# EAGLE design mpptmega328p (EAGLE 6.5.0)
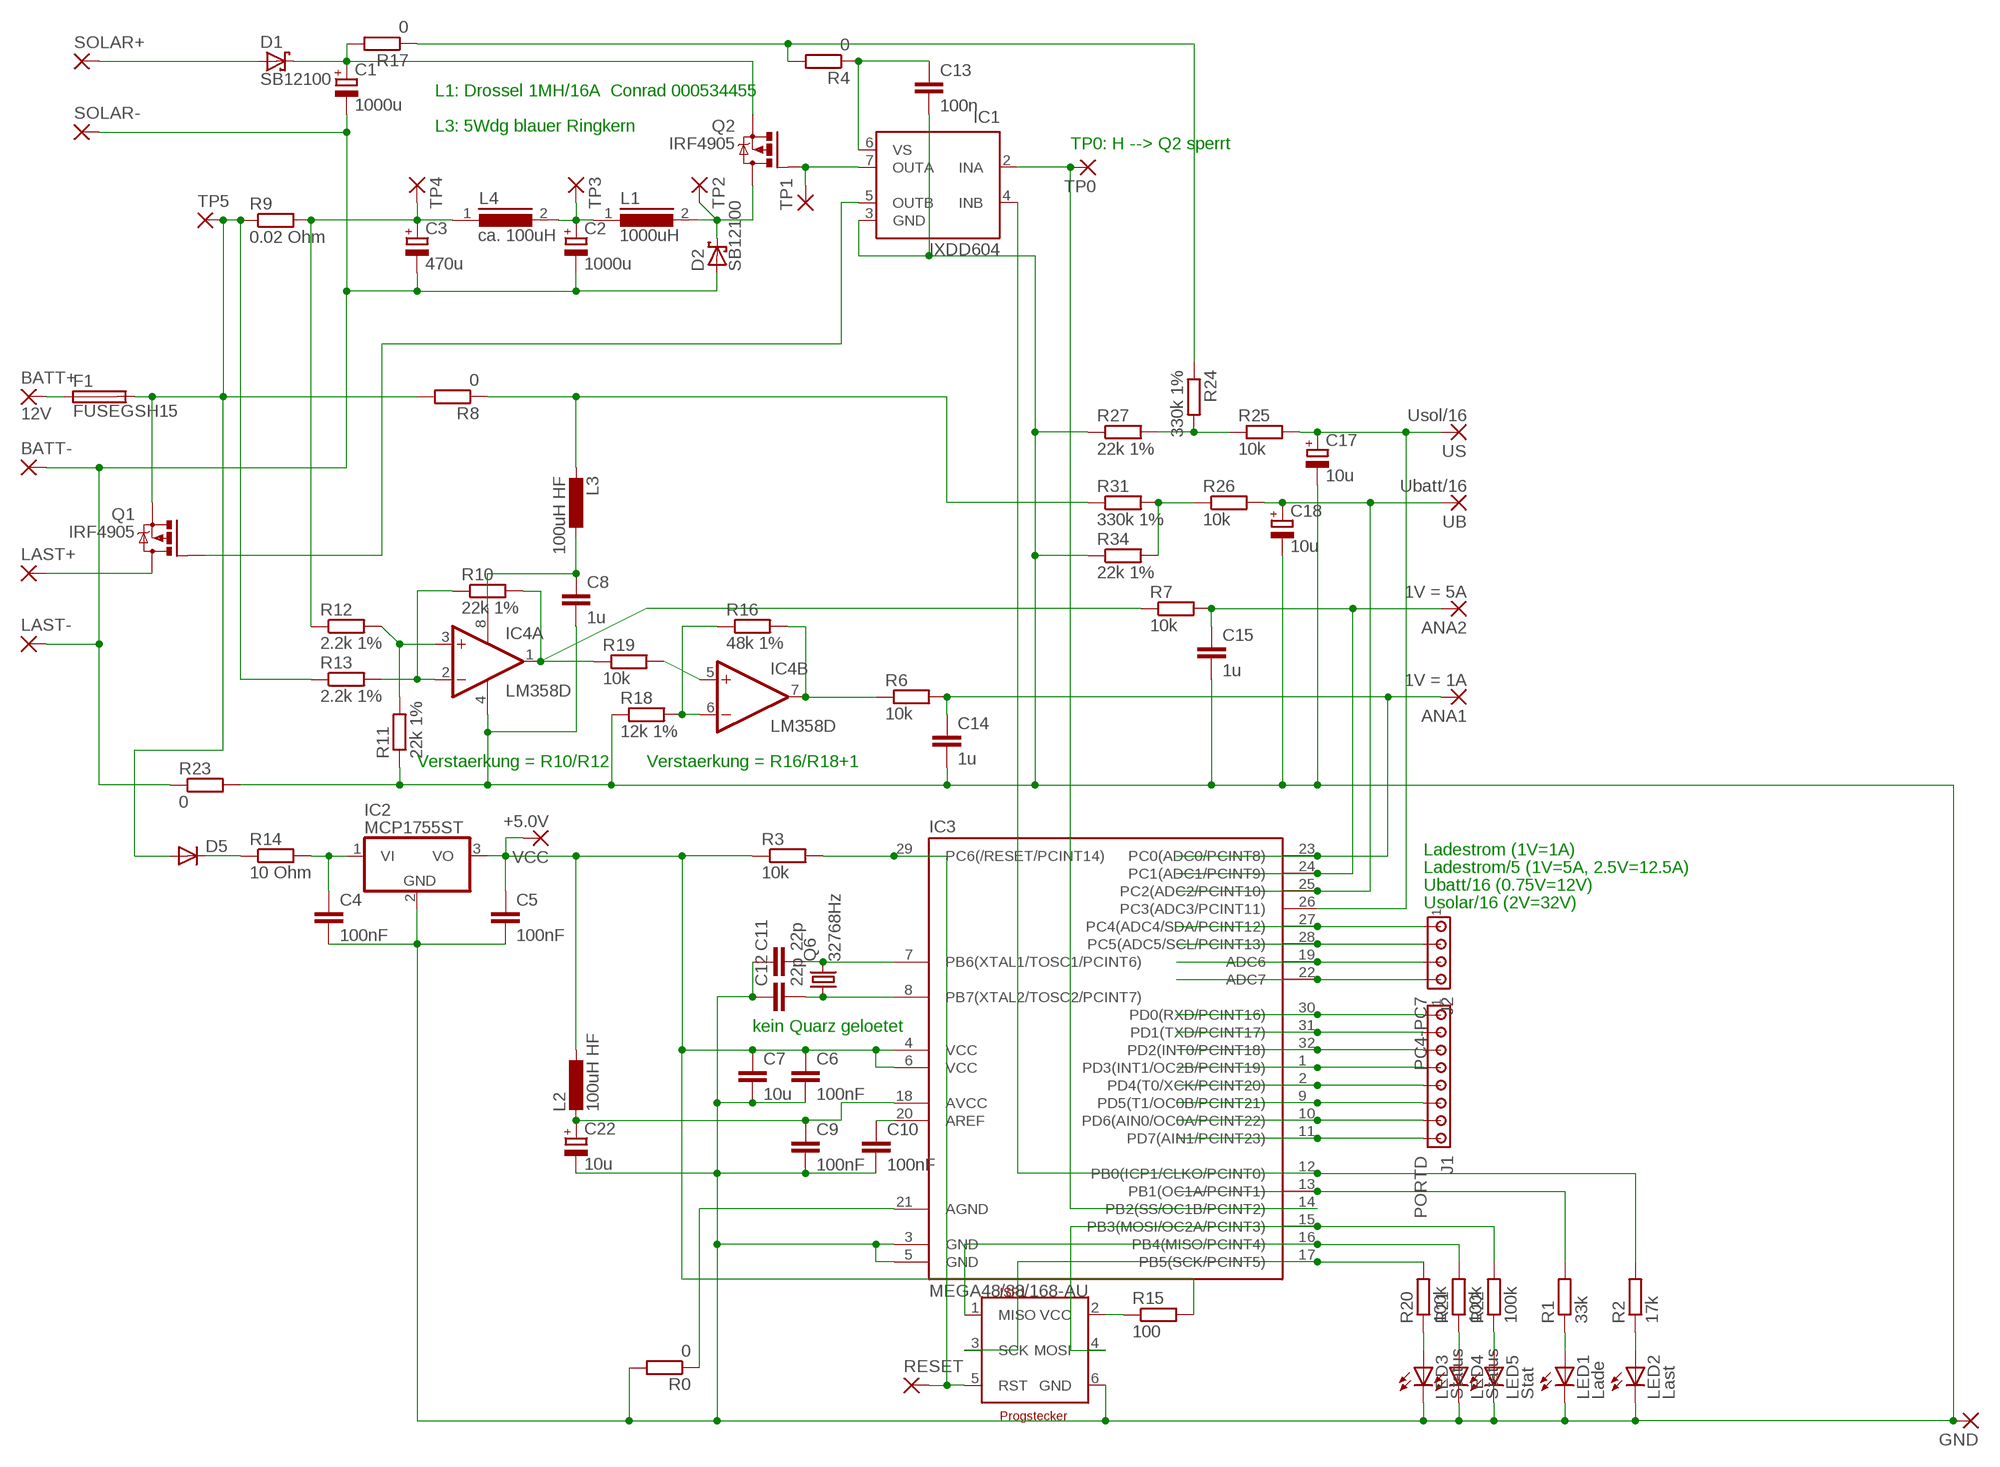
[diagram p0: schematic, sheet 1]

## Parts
ANA1  1V = 1A  WIREPAD1,6/0,8  [1,6/0,8]
ANA2  1V = 5A  WIREPAD1,6/0,8  [1,6/0,8]
BATT+  12V  WIREPAD3,81/1,1  [3,81/1,1]
BATT-  WIREPAD3,81/1,1  [3,81/1,1]
C1  1000u  CPOL-EUE5-13  [E5-13]
C2  1000u  CPOL-EUE5-13  [E5-13]
C3  470u  CPOL-EUE3.5-10  [E3,5-10]
C4  100nF  C-EUC1206  [C1206]
C5  100nF  C-EUC1206  [C1206]
C6  100nF  C-EUC1206K  [C1206K]
C7  10u  C-EUC1206  [C1206]
C8  1u  C-EUC1206K  [C1206K]
C9  100nF  C-EUC1206K  [C1206K]
C10  100nF  C-EUC1206K  [C1206K]
C11  22p  C-EU025-024X044  [C025-024X044]
C12  22p  C-EU025-024X044  [C025-024X044]
C13  100n  C-EUC1206K  [C1206K]
C14  1u  C-EU025-025X050  [C025-025X050]
C15  1u  C-EU025-025X050  [C025-025X050]
C17  10u  CPOL-EUE2-5  [E2-5]
C18  10u  CPOL-EUE2-5  [E2-5]
C22  10u  CPOL-EUE2.5-5  [E2,5-5]
D1  SB12100  1N5908  [C4111-15]
D2  SB12100  1N5908  [C4111-15]
D5  1N4004  [DO41-10]
F1  FUSEGSH15  [GSH15]
GND  WIREPAD2,15/1,0  [2,15/1,0]
IC1  IXDD604  IR4427S  [SO08]
IC2  MCP1755ST  MCP1703DB  [SOT223]
IC3  MEGA48/88/168-AU  [TQFP32-08]
IC4  LM358D  [SO08]
ISP1  Progstecker  ISP6N  [ISP6]
J1  PORTD  MTA08-100  [10X08MTA]
J2  PC4-PC7  MTA04-100  [10X04MTA]
L1  1000uH  A26GFC  [A26GFC]
L2  100uH HF  L-EU0204/7  [0204/7]
L3  100uH HF  L-EU0204/7  [0204/7]
L4  ca. 100uH  82114R  [82114R]
LAST+  WIREPAD3,81/1,1  [3,81/1,1]
LAST-  WIREPAD3,81/1,1  [3,81/1,1]
LED1  Lade  LEDSFH482  [SFH482]
LED2  Last  LEDSFH482  [SFH482]
LED3  Status  LEDSFH482  [SFH482]
LED4  Status  LEDSFH482  [SFH482]
LED5  Stat  LEDSFH482  [SFH482]
Q1  IRF4905  IRF9530  [TO220BV]
Q2  IRF4905  IRF9530  [TO220BV]
Q6  32768Hz  CRYSTALTC26V  [TC26V]
R0  0  R-EU_R1206  [R1206]
R1  33k  R-EU_0204/2V  [0204V@1]
R2  17k  R-EU_0204/2V  [0204V@1]
R3  10k  R-EU_M1406  [M1406]
R4  0  R-EU_R1206  [R1206]
R6  10k  R-EU_0204/2V  [0204V@1]
R7  10k  R-EU_0204/2V  [0204V@1]
R8  0  R-EU_R1206  [R1206]
R9  0.02 Ohm  R-EU_0204/7  [0204/7@1]
R10  22k 1%  R-EU_0204/2V  [0204V@1]
R11  22k 1%  R-EU_0204/2V  [0204V@1]
R12  2.2k 1%  R-EU_0204/7  [0204/7@1]
R13  2.2k 1%  R-EU_0204/7  [0204/7@1]
R14  10 Ohm  R-EU_0204/5  [0204/5@1]
R15  100  R-EU_0204/5  [0204/5@1]
R16  48k 1%  R-EU_0204/2V  [0204V@1]
R17  0  R-EU_R1206  [R1206]
R18  12k 1%  R-EU_0204/5  [0204/5@1]
R19  10k  R-EU_0204/5  [0204/5@1]
R20  100k  R-EU_0204/2V  [0204V@1]
R21  100k  R-EU_0204/2V  [0204V@1]
R22  100k  R-EU_0204/2V  [0204V@1]
R23  0  R-EU_R1206  [R1206]
R24  330k 1%  R-EU_0204/7  [0204/7@1]
R25  10k  R-EU_0204/5  [0204/5@1]
R26  10k  R-EU_0204/5  [0204/5@1]
R27  22k 1%  R-EU_0204/5  [0204/5@1]
R31  330k 1%  R-EU_0204/7  [0204/7@1]
R34  22k 1%  R-EU_0204/5  [0204/5@1]
RESET  WIREPAD1,6/0,8  [1,6/0,8]
SOLAR+  WIREPAD3,81/1,1  [3,81/1,1]
SOLAR-  WIREPAD3,81/1,1  [3,81/1,1]
TP0  WIREPAD1,6/0,8  [1,6/0,8]
TP1  WIREPAD2,15/1,0  [2,15/1,0]
TP2  WIREPAD2,15/1,0  [2,15/1,0]
TP3  WIREPAD2,15/1,0  [2,15/1,0]
TP4  WIREPAD2,15/1,0  [2,15/1,0]
TP5  WIREPAD2,15/1,0  [2,15/1,0]
UB  Ubatt/16  WIREPAD2,15/1,0  [2,15/1,0]
US  Usol/16  WIREPAD2,15/1,0  [2,15/1,0]
VCC  +5.0V  WIREPAD2,54/0,9  [2,54/0,9]

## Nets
AGND [duenn]: IC3.21(AGND) R0.1
AVCC [duenn]: C9.1 C22.+ IC3.18(AVCC) L2.2
GND [dick]: C4.2 C5.2 C6.2 C7.2 C8.2 C9.2 C10.2 C11.1 C12.1 C13.2 C14.2 C15.2 C17.- C18.- C22.- GND.1(P) IC1.3(GND) IC2.2(GND) IC3.3(GND) IC3.5(GND) IC4.4(P:V-) ISP1.6(GND) LED1.K(C) LED2.K(C) LED3.K(C) LED4.K(C) LED5.K(C) R0.2 R11.1 R18.1 R23.2 R27.1 R34.1
GND2 [sehrdick]: BATT-.1(P) C1.- C2.- C3.- D2.A LAST-.1(P) R23.1 SOLAR-.1(P)
N$1 [dick]: LED1.A R1.1
N$2: IC1.4(INB) IC3.12(PB0(ICP1/CLKO/PCINT0)) R2.2
N$3: IC3.17(PB5(SCK/PCINT5)) ISP1.3(SCK) R20.2
N$4: IC3.13(PB1(OC1A/PCINT1)) R1.2
N$5 [dick]: LED2.A R2.1
N$6 [duenn]: C17.+ IC3.26(PC3(ADC3/PCINT11)) R25.2 US.1(P)
N$7: IC1.2(INA) IC3.14(PB2(SS/OC1B/PCINT2)) TP0.1(P)
N$8 [duenn]: IC1.5(OUTB) Q1.G
N$9 [duenn]: C18.+ IC3.25(PC2(ADC2/PCINT10)) R26.2 UB.1(P)
N$10: C10.1 IC3.20(AREF)
N$11: ISP1.2(VCC) R15.1
N$12 [duenn]: ANA2.1(P) C15.1 IC3.24(PC1(ADC1/PCINT9)) R7.2
N$13 [duenn]: ANA1.1(P) C14.1 IC3.23(PC0(ADC0/PCINT8)) R6.2
N$14 [dick]: D5.C R14.1
N$15: IC3.27(PC4(ADC4/SDA/PCINT12)) J2.1
N$16: IC3.28(PC5(ADC5/SCL/PCINT13)) J2.2
N$17: IC3.19(ADC6) J2.3
N$18 [dick]: C4.1 IC2.1(VI) R14.2
N$19: IC3.22(ADC7) J2.4
N$20 [sehrdick]: BATT+.1(P) F1.1
N$21 [sehrdick]: D1.A SOLAR+.1(P)
N$24 [sehrdick]: D2.C L1.2 Q2.D TP2.1(P)
N$25: IC3.16(PB4(MISO/PCINT4)) ISP1.1(MISO) R21.2
N$26: IC3.29(PC6(/RESET/PCINT14)) ISP1.5(RST) R3.2 RESET.1(P)
N$27: IC3.15(PB3(MOSI/OC2A/PCINT3)) ISP1.4(MOSI) R22.2
N$28 [dick]: IC1.7(OUTA) Q2.G TP1.1(P)
N$29 [sehrdick]: C2.+ L1.1 L4.2 TP3.1(P)
N$31 [dick]: LED3.A R20.1
N$32 [duenn]: IC4.2(A:-IN) R10.1 R13.2
N$33 [dick]: LED4.A R21.1
N$34 [dick]: LED5.A R22.1
N$35: C11.2 IC3.7(PB6(XTAL1/TOSC1/PCINT6)) Q6.2
N$36: C12.2 IC3.8(PB7(XTAL2/TOSC2/PCINT7)) Q6.1
N$37 [duenn]: IC4.3(A:+IN) R11.2 R12.2
N$38 [dick]: L3.2 R8.1 R31.1
N$39 [duenn]: IC4.6(B:-IN) R16.1 R18.2
N$40 [duenn]: IC4.5(B:+IN) R19.2
N$42 [duenn]: IC4.7(B:OUT) R6.1 R16.2
N$43 [sehrdick]: LAST+.1(P) Q1.D
N$47 [duenn]: IC4.1(A:OUT) R7.1 R10.2 R19.1
N$50: IC3.30(PD0(RXD/PCINT16)) J1.1
N$51: IC3.31(PD1(TXD/PCINT17)) J1.2
N$52: IC3.32(PD2(INT0/PCINT18)) J1.3
N$53: IC3.1(PD3(INT1/OC2B/PCINT19)) J1.4
N$54: IC3.2(PD4(T0/XCK/PCINT20)) J1.5
N$55: IC3.9(PD5(T1/OC0B/PCINT21)) J1.6
N$56: IC3.10(PD6(AIN0/OC0A/PCINT22)) J1.7
N$57: IC3.11(PD7(AIN1/PCINT23)) J1.8
N$58 [duenn]: R24.2 R25.1 R27.2
N$60 [sehrdick]: C3.+ L4.1 R9.2 R12.1 TP4.1(P)
N$64 [duenn]: R26.1 R31.2 R34.2
SOLARDUENN [dick]: R4.2 R17.1 R24.1
SOLPLUS [sehrdick]: C1.+ D1.C Q2.S R17.2
V12 [sehrdick]: D5.A F1.2 Q1.S R8.2 R9.1 R13.1 TP5.1(P)
V+ [dick]: C8.1 IC4.8(P:V+) L3.1
VCC [duenn]: C5.1 C6.1 C7.1 IC2.3(VO) IC3.4(VCC) IC3.6(VCC) L2.1 R3.1 R15.2 VCC.1(P)
VS [dick]: C13.1 IC1.6(VS) R4.1

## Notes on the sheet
- L1: Drossel 1MH/16A  Conrad 000534455
- L3: 5Wdg blauer Ringkern
- TP0: H --> Q2 sperrt
- Verstaerkung = R10/R12 | Verstaerkung = R16/R18+1
- Ladestrom (1V=1A)
- Ladestrom/5 (1V=5A, 2.5V=12.5A)
- Ubatt/16 (0.75V=12V)
- Usolar/16 (2V=32V)
- kein Quarz geloetet

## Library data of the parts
ANA1 ANA2 BATT+ BATT- GND LAST+ LAST- RESET SOLAR+ SOLAR- TP0 TP1-TP5 UB US VCC = wirepad:WIREPAD: Wire PAD connect wire on PCB
C1-C3 C17 C18 C22 = rcl:CPOL-EU: POLARIZED CAPACITOR, European symbol
C4-C15 = rcl:C-EU: CAPACITOR, European symbol
D1 D2 = diode:1N5908: DIODE
D5 = diode:1N4004: DIODE
F1 = fuse:FUSE: Fuse; OC_FARNELL: unknown; OC_NEWARK: unknown
IC1 = ir:IR4427: DUAL LOW SIDE DRIVER Source: ID4426.pdf; MF: INTERNATIONAL RECTIFIER(IR); MPN: IR4427STRPBF; OC_FARNELL: 8639094; OC_NEWARK: 63J7933
IC2 = linear:MCP1703: 250 mA, 16V, Low Quiescent Current LDO Regulator Source: http://ww1.microchip.com/downloads/en/DeviceDoc/22049b.pdf
IC3 = avr-7:MEGA48/88/168
IC4 = linear:LM358: OP AMP also LM158; LM258; LM2904 Source: http://cache.national.com/ds/LM/LM158.pdf
ISP1 = stecker:ISP6: ISP-Stecker 6polig
J1 = con-amp:MTA08-100: AMP connector
J2 = con-amp:MTA04-100: AMP connector
L1 = inductors:A26GFC: INDUCTOR
L2 L3 = rcl:L-EU: INDUCTOR, European symbol
L4 = inductors:82114R: INDUCTOR
LED1-LED5 = led:LED: LED
Q1 Q2 = transistor-power:IRF9530: P-CHANNEL HEXFET POWER-MOS-FET Source: http://www.irf.com/product-info/datasheets/data/irf9530.pdf
Q6 = crystal:CRYSTAL: CRYSTAL; OC_FARNELL: unknown; OC_NEWARK: unknown
R0 R1-R4 R6-R27 R31 R34 = rcl:R-EU_: RESISTOR, European symbol

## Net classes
1 dick: width 0.508 mm, clearance 0.203 mm
2 sehrdick: width 2.032 mm, clearance 0.508 mm
3 duenn: width 0.381 mm

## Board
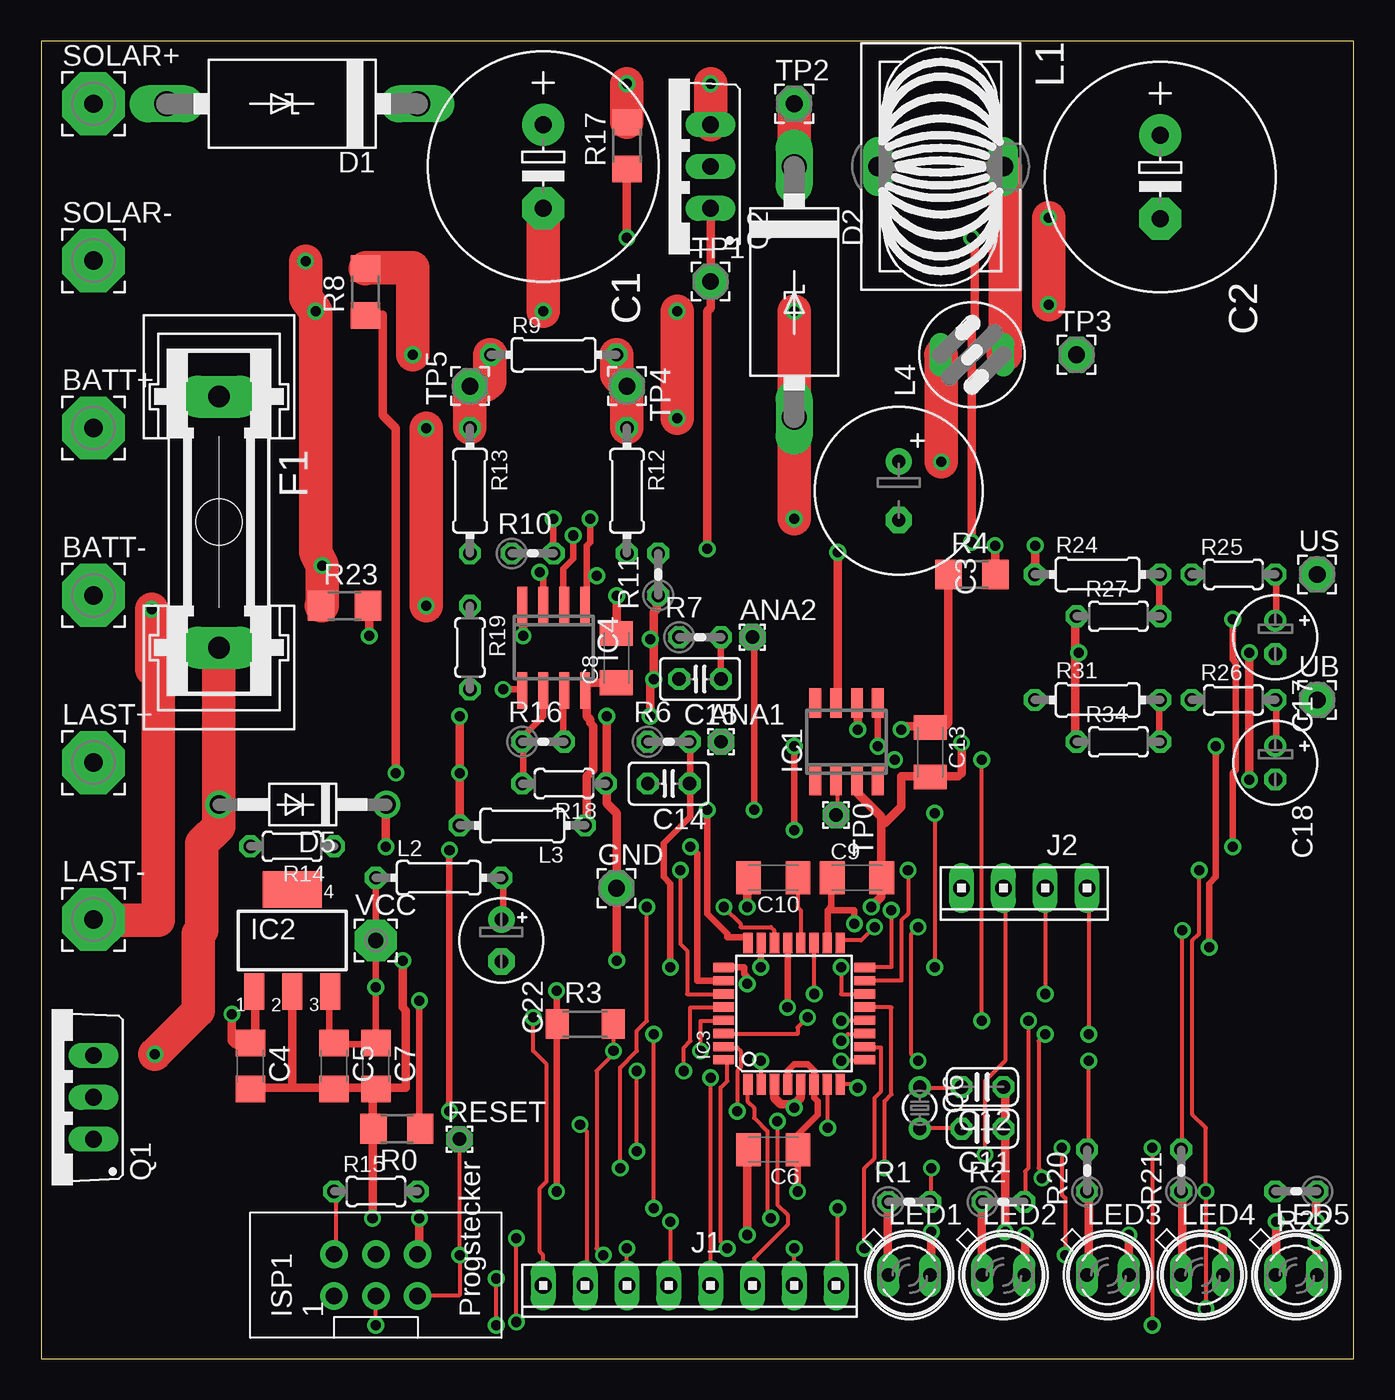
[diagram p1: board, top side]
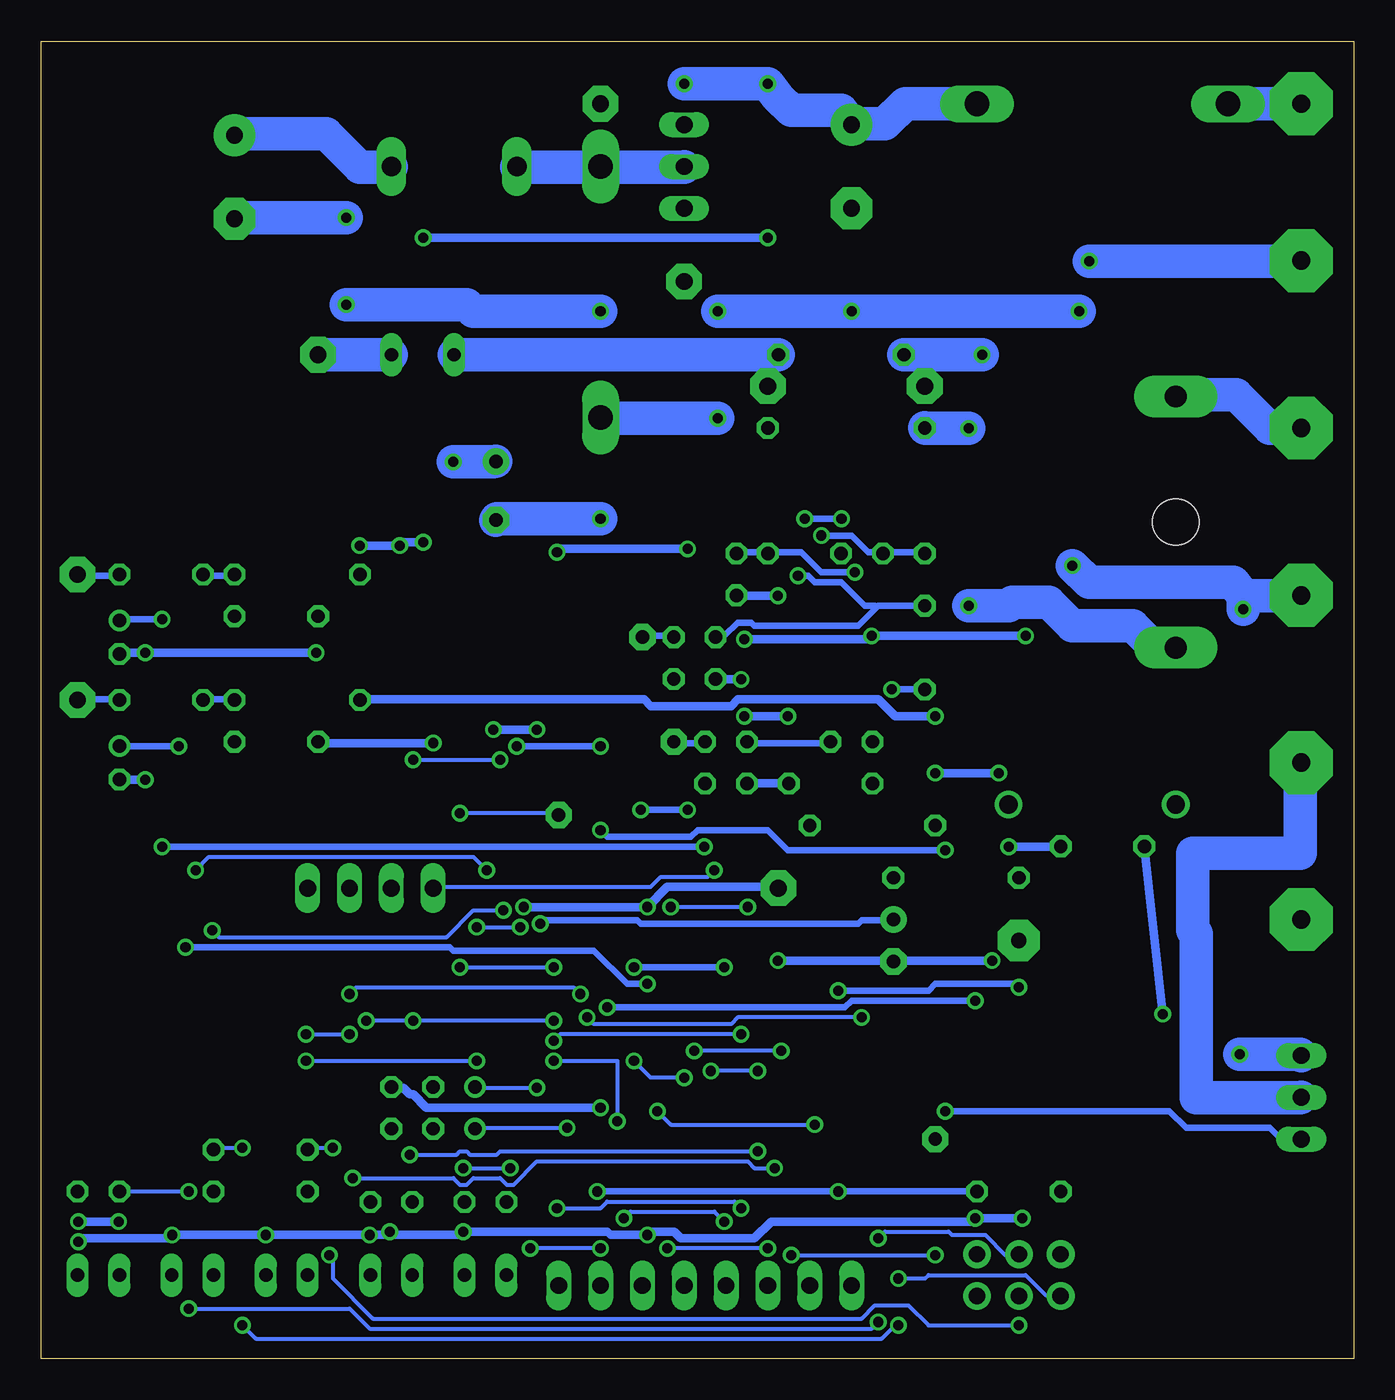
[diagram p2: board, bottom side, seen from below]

Size 79.68 x 80 mm. Coordinates in mm from the lower left corner, seen from the top.
Outline: 0,0 79.68,0 79.68,80 0,80 0,0
Copper layers (1*16): Top 0.035mm / dielectric 1.5mm / Bottom 0.035mm
Design rules "default": minimum track width 10mil, minimum drill 24mil, track to track 8mil, track to pad 8mil, pad to pad 8mil, via to via 8mil, smd to smd 8mil, copper to edge 40mil, drill to drill 8mil, minimum pad ring 10mil, minimum via ring 8mil, stop-mask expansion 4mil, vias tented up to drill 0mil, thermal gap 10mil

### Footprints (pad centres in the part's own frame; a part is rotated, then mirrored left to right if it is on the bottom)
1,6/0,8 = drill 0.813 pad 1.6 octagon: 1 0,0
3,81/1,1 = drill 1.118 pad 3.81 octagon: 1 0,0
E5-13 = drill 1.016 pad 2.54: + -2.54,0 | drill 1.016 pad 2.54 octagon: - 2.54,0
E3,5-10 = drill 0.813 pad 1.6: + -1.778,0 | drill 0.813 pad 1.6 octagon: - 1.778,0
C1206 = smd 1.6 x 1.8: 1 -1.4,0; 2 1.4,0
C1206K = smd 1.5 x 2: 1 -1.5,0; 2 1.5,0
C025-024X044 = drill 0.813 octagon: 1 -1.27,0; 2 1.27,0
C025-025X050 = drill 0.813 octagon: 1 -1.27,0; 2 1.27,0
E2-5 = drill 0.813 pad 1.27: + -1.016,0 | drill 0.813 pad 1.27 octagon: - 1.016,0
E2,5-5 = drill 0.813 pad 1.6: + -1.27,0 | drill 0.813 pad 1.6 octagon: - 1.27,0
C4111-15 = drill 1.499 long: A 7.62,0; C -7.62,0
DO41-10 = drill 1.118: A 5.08,0; C -5.08,0
GSH15 = drill 1.321 pad 2.54 long: 1 -7.62,0; 2 7.62,0 | hole 2.794: 0,0
2,15/1,0 = drill 1.016 pad 2.159 octagon: 1 0,0
SO08 = smd 0.72 x 1.78: 1 -1.905,-2.35; 2 -0.635,-2.35; 3 0.635,-2.35; 4 1.905,-2.35; 5 1.905,2.35; 6 0.635,2.35; 7 -0.635,2.35; 8 -1.905,2.35
SOT223 = smd 1.219 x 2.235: 1 -2.311,-3.099; 2 0,-3.099; 3 2.311,-3.099 | smd 3.6 x 2.2: 4 0,3.099
TQFP32-08 = smd 1.27 x 0.559: 1 -4.293,2.8; 2 -4.293,2; 3 -4.293,1.2; 4 -4.293,0.4; 5 -4.293,-0.4; 6 -4.293,-1.2; 7 -4.293,-2; 8 -4.293,-2.8; 17 4.293,-2.8; 18 4.293,-2; 19 4.293,-1.2; 20 4.293,-0.4; 21 4.293,0.4; 22 4.293,1.2; 23 4.293,2; 24 4.293,2.8 | smd 0.559 x 1.27: 9 -2.8,-4.293; 10 -2,-4.293; 11 -1.2,-4.293; 12 -0.4,-4.293; 13 0.4,-4.293; 14 1.2,-4.293; 15 2,-4.293; 16 2.8,-4.293; 25 2.8,4.293; 26 2,4.293; 27 1.2,4.293; 28 0.4,4.293; 29 -0.4,4.293; 30 -1.2,4.293; 31 -2,4.293; 32 -2.8,4.293
SO08' = smd 0.6 x 2.2: 1 -1.905,-2.6; 2 -0.635,-2.6; 3 0.635,-2.6; 4 1.905,-2.6; 5 1.905,2.6; 6 0.635,2.6; 7 -0.635,2.6; 8 -1.905,2.6
ISP6 = drill 1 pad 1.676: 1 -1.27,2.54; 2 1.27,2.54; 3 -1.27,0; 4 1.27,0; 5 -1.27,-2.54; 6 1.27,-2.54
10X08MTA = drill 1.016 long: 1 8.89,0; 2 6.35,0; 3 3.81,0; 4 1.27,0; 5 -1.27,0; 6 -3.81,0; 7 -6.35,0; 8 -8.89,0
10X04MTA = drill 1.016 long: 1 3.81,0; 2 1.27,0; 3 -1.27,0; 4 -3.81,0
A26GFC = drill 1.194 long: 1 0,3.81; 2 0,-3.81
0204/7 = drill 0.813 octagon: 1 -3.81,0; 2 3.81,0
82114R = drill 0.813 long: 1 0,1.905; 2 0,-1.905
SFH482 = drill 0.813 long: A -1.27,0; K 1.27,0
TO220BV = drill 1.016 long: D 0,-2.54; G -2.54,-2.54; S 2.54,-2.54
TC26V = drill 0.813: 1 -1.27,0; 2 1.27,0
R1206 = smd 1.6 x 1.803: 1 -1.422,0; 2 1.422,0
0204V@1 = drill 0.813 octagon: 1 -1.27,0; 2 1.27,0
M1406 = smd 1.4 x 1.8: 1 -1.7,0; 2 1.7,0
0204/7@1 = drill 0.813 octagon: 1 -3.81,0; 2 3.81,0
0204/5@1 = drill 0.813 octagon: 1 -2.54,0; 2 2.54,0
2,54/0,9 = drill 0.914 pad 2.54 octagon: 1 0,0

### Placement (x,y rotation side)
ANA1  41.27,37.47 0 top
ANA2  43.18,43.81 0 top
BATT+  3.17,56.52 0 top
BATT-  3.17,46.35 0 top
C1  30.48,72.39 270 top
C2  67.94,71.75 270 top
C3  52.07,52.7 270 top
C4  12.7,17.78 270 top
C5  17.78,17.78 270 top
C6  44.45,12.7 180 top
C7  20.32,17.78 270 top
C8  34.92,42.55 90 top
C9  49.53,29.21 0 top
C10  44.45,29.21 180 top
C11  57.15,13.97 180 top
C12  57.15,16.51 180 top
C13  53.98,36.83 270 top
C14  38.1,34.92 180 top
C15  40.01,41.27 180 top
C17  74.93,43.81 270 top
C18  74.93,36.2 270 top
C22  27.94,25.4 270 top
D1  15.24,76.2 180 top
D2  45.72,64.77 270 top
D5  15.88,33.66 180 top
F1  10.79,50.8 270 top
GND  34.92,28.57 0 top
IC1  48.9,37.47 0 top
IC2  15.24,25.4 0 top
IC3  45.72,20.95 90 top
IC4  LM358D  [SO08']  31.11,43.18 180 top
ISP1  20.32,5.08 90 top
J1  39.37,4.45 180 top
J2  59.69,28.57 180 top
L1  54.61,72.39 270 top
L2  24.13,29.21 0 top
L3  29.21,32.38 180 top
L4  56.52,60.96 90 top
LAST+  3.17,36.2 0 top
LAST-  3.17,26.67 0 top
LED1  52.7,5.08 0 top
LED2  58.42,5.08 0 top
LED3  64.77,5.08 0 top
LED4  70.48,5.08 0 top
LED5  76.2,5.08 0 top
Q1  0.64,15.88 90 top
Q2  38.1,72.39 90 top
Q6  53.34,15.24 270 top
R0  21.59,13.97 180 top
R1  52.7,9.53 0 top
R2  58.42,9.53 0 top
R3  33.02,20.32 0 top
R4  56.52,47.62 0 top
R6  38.1,37.47 0 top
R7  40.01,43.81 0 top
R8  19.68,64.77 90 top
R9  31.11,60.96 0 top
R10  29.84,48.9 0 top
R11  37.47,47.62 90 top
R12  35.56,52.7 270 top
R13  26.04,52.7 270 top
R14  15.24,31.11 180 top
R15  20.32,10.16 0 top
R16  30.48,37.47 0 top
R17  35.56,73.66 90 top
R18  31.75,34.92 180 top
R19  26.04,43.18 270 top
R20  63.5,11.43 90 top
R21  69.22,11.43 90 top
R22  76.2,10.16 180 top
R23  18.41,45.72 0 top
R24  64.14,47.62 0 top
R25  72.39,47.62 0 top
R26  72.39,40.01 0 top
R27  65.41,45.09 0 top
R31  64.14,40.01 0 top
R34  65.41,37.47 0 top
RESET  25.4,13.34 0 top
SOLAR+  3.17,76.2 0 top
SOLAR-  3.17,66.67 0 top
TP0  48.26,33.02 270 top
TP1  40.64,65.41 0 top
TP2  45.72,76.2 0 top
TP3  62.87,60.96 0 top
TP4  35.56,59.05 270 top
TP5  26.04,59.05 90 top
UB  77.47,40.01 0 top
US  77.47,47.62 0 top
VCC  20.32,25.4 0 top

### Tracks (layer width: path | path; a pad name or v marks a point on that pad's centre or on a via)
AGND  (via drill 0.61)
  Top 0.381: v45.31,21.34 45.31,25.2 IC3.21 | v22.96,21.74 22.96,14.02 R0.1
  Bottom 0.381: v45.31,21.34 30.89,21.34 30.48,21.74 v22.96,21.74
AVCC  (via drill 0.61)
  Top 0.381: 47.85,27.33 47.95,27.43 47.95,29.06 C9.1 | 47.85,27.33 47.75,27.23 47.75,25.4 IC3.18 | L2.2 28.04,29.06 28.04,26.82 C22.+ | v49.38,26.42 49.38,27.23 47.95,27.23 47.85,27.33
  Bottom 0.381: v49.38,26.42 49.17,26.62 43.48,26.62 43.28,26.42 30.07,26.42 29.87,26.62 28.04,26.62 C22.+
GND  (via drill 0.61)
  Top 0.508: 45.72,15.44 44.91,15.44 44.5,15.85 44.5,16.66 IC3.3 | 45.72,15.44 46.13,15.85 IC3.5 | v45.72,15.24 45.72,15.44 | C12.1 58.52,16.46 58.52,14.02 C11.1 58.52,13.82 v58.52,7.72 | v42.88,7.52 42.88,12.6 C6.2 | v54.05,7.72 54.05,5.08 LED1.K | v59.74,7.52 59.74,5.08 LED2.K | v66.04,7.52 LED3.K | v71.73,7.52 71.73,5.08 LED4.K | v77.42,7.11 77.42,5.08 LED5.K | 15.24,16.46 12.8,16.46 C4.2 | IC2.2 15.24,16.46 | C7.2 20.32,16.46 17.88,16.46 C5.2 17.68,16.46 15.24,16.46 | C7.2 20.12,16.26 20.12,14.02 R0.2 20.12,13.82 v20.12,8.53 | v22.96,8.53 22.96,6.5 ISP1.6 | v34.95,24.18 34.95,28.45 GND.1 34.95,28.65 34.95,33.12 34.34,33.73 34.34,34.75 R18.1 34.34,35.15 v34.34,39.01 | v42.88,27.43 42.88,29.06 C10.2 | v50.39,27.43 51,28.04 51,29.06 C9.2 51,29.46 51,32.51 | v21.95,24.18 21.95,21.34 22.15,21.13 22.15,16.46 20.52,16.46 C7.2 | v34.95,46.33 34.95,44.09 C8.2 | 37.19,43.69 37.19,45.31 37.39,45.52 37.39,46.33 R11.1 | 37.19,43.69 v37.19,41.25 36.98,41.25 v36.98,39.01 | v19.91,43.89 19.91,45.72 R23.2 | v29.26,43.89 29.26,45.72 IC4.4 | v36.98,43.69 37.19,43.69 | v73.36,42.88 v73.36,35.15 | 62.79,42.88 62.79,44.91 R27.1 | 62.79,42.88 62.79,37.59 R34.1 | 51,32.51 51,32.92 49.58,34.34 49.58,34.95 IC1.3 | 51,32.51 51.21,32.51 52.22,33.53 52.22,35.36 53.85,35.36 C13.2 54.05,35.36 55.68,35.36 55.88,35.56 v55.88,37.39 | v62.99,42.88 62.79,42.88
  Bottom 0.508: v45.72,15.24 56.29,15.24 57.1,16.05 57.3,16.05 57.71,16.46 58.32,16.46 C12.1 | 58.52,7.52 54.05,7.52 v54.05,7.72 45.31,7.72 45.11,7.52 v42.88,7.52 42.88,7.72 41.25,7.72 40.84,7.32 36.37,7.32 35.36,8.33 22.96,8.33 v22.96,8.53 v20.12,8.53 | 58.52,7.52 v59.74,7.52 v66.04,7.52 v71.73,7.52 71.73,7.32 77.22,7.32 v77.42,7.11 | v58.52,7.72 58.52,7.52 | v34.95,24.18 28.04,24.18 C22.- 27.84,24.18 v21.95,24.18 | GND.1 34.95,28.65 41.66,28.65 v42.88,27.43 v50.39,27.43 | v34.95,46.33 37.39,46.33 R11.1 | v37.19,41.25 38.61,41.25 C15.2 | v19.91,43.89 v29.26,43.89 29.26,43.69 v36.98,43.69 | v73.36,35.15 74.78,35.15 C18.- | C17.- 74.78,42.88 v73.36,42.88 v62.99,42.88 | R18.1 34.34,34.95 36.78,34.95 C14.2 | v55.88,37.39 62.79,37.39 R34.1 | v34.34,39.01 v36.98,39.01
GND2  (via drill 0.61)
  Top 2.032: v45.72,51 D2.A v45.72,63.6 | v61.16,64.01 v61.16,69.29 | v6.71,45.52 6.71,41.86 7.11,41.45 7.11,26.62 3.25,26.62 LAST-.1 | R23.1 17.07,45.72 v17.07,48.16 16.66,48.97 v16.66,63.6 16.05,64.41 v16.05,66.65 | v30.48,63.6 C1.- | v38.61,57.1 v38.61,63.6
  Bottom 2.032: v45.72,51 52.02,51 C3.- | v61.16,69.29 67.87,69.29 C2.- | v61.16,64.01 53.85,64.01 53.44,63.6 v45.72,63.6 | 6.71,46.33 3.25,46.33 BATT-.1 | v6.71,45.52 6.71,46.33 | v17.07,48.16 16.05,47.14 7.32,47.14 6.71,46.33 | v38.61,63.6 v30.48,63.6 v16.66,63.6 | v38.61,57.1 45.72,57.1 D2.A | v16.05,66.65 3.25,66.65 SOLAR-.1
N$1
  Top 0.508: LED1.A 51.41,5.08 51.41,9.35 R1.1
N$2  (via drill 0.61)
  Top 0.254: v59.94,20.52 59.94,11.58 59.74,11.38 59.74,9.55 R2.2 | v48.56,20.52 49.99,20.52 IC3.12 | IC1.4 50.8,35.56 51.61,36.37 v51.82,36.37 | v57.1,20.52 v57.1,36.37
  Bottom 0.254: v48.56,20.52 v57.1,20.52 v59.94,20.52 | v57.1,36.37 v51.82,36.37
N$3  (via drill 0.61)
  Top 0.254: v50.6,26.21 49.78,25.4 48.56,25.4 IC3.17 | v53.24,26.21 52.83,25.81 52.83,18.49 v53.24,18.09 | v63.6,18.09 63.6,12.8 R20.2 | v20.32,2.03 ISP1.3 | v62.18,6.3 62.18,9.75 61.98,9.96 v61.98,12.8
  Bottom 0.254: v53.24,26.21 v50.6,26.21 | v63.6,18.09 v53.24,18.09 | v20.32,2.03 25.81,2.03 27.03,3.25 29.06,3.25 29.87,2.44 59.54,2.44 61.98,4.88 61.98,6.3 v62.18,6.3 | v61.98,12.8 63.4,12.8 R20.2
N$4  (via drill 0.61)
  Top 0.254: v51.21,11.58 51.21,15.65 51.61,16.05 51.61,21.34 50.19,21.34 IC3.13 | v54.05,11.58 54.05,9.55 R1.2
  Bottom 0.254: v54.05,11.58 v51.21,11.58
N$5
  Top 0.508: LED2.A 57.1,5.08 57.1,9.35 R2.1
N$6  (via drill 0.61)
  Top 0.381: C17.+ 74.98,44.91 74.98,47.55 R25.2 | v39.42,31.09 39.83,30.68 39.83,22.96 41.25,22.96 IC3.26 | v72.34,31.09 72.34,35.56 72.54,35.76 72.54,42.27 72.34,42.47 v72.34,44.91
  Bottom 0.381: R25.2 74.98,47.55 77.42,47.55 US.1 | v72.34,31.09 v39.42,31.09 | v72.34,44.91 74.78,44.91 C17.+
N$7  (via drill 0.61)
  Top 0.254: IC1.2 48.36,34.95 48.36,33.12 TP0.1 | v48.56,23.77 48.56,22.15 49.99,22.15 IC3.14 | v54.25,33.12 v54.25,23.77
  Bottom 0.254: v54.25,23.77 v48.56,23.77 | v54.25,33.12 48.36,33.12 TP0.1
N$8  (via drill 0.61)
  Top 0.381: v50.8,37.19 IC1.5 | v45.72,32.11 v45.72,37.19 | v24.79,15.04 v24.79,30.89
  Bottom 0.381: v45.72,37.19 v50.8,37.19 | v45.72,32.11 45.31,31.7 40.23,31.7 39.83,32.11 35.56,32.11 34.34,30.89 v24.79,30.89 | v24.79,15.04 11.18,15.04 10.16,14.02 5.08,14.02 4.47,13.41 3.25,13.41 Q1.G
N$9  (via drill 0.61)
  Top 0.381: C18.+ 74.98,37.39 74.98,39.83 R26.2 | v42.88,22.76 42.88,23.16 42.67,23.37 42.67,23.77 41.45,23.77 IC3.25 | v70.92,24.99 70.92,28.85 71.32,29.26 v71.32,37.19
  Bottom 0.381: v42.88,22.76 44.09,22.76 46.13,24.79 54.66,24.79 54.86,24.99 v70.92,24.99 | v71.32,37.19 74.78,37.19 C18.+ | UB.1 77.42,40.03 74.98,40.03 R26.2
N$10
  Top 0.254: C10.1 45.92,29.06 45.92,27.43 46.13,27.23 46.13,25.4 IC3.20
N$11
  Top 0.254: ISP1.2 17.88,6.5 17.88,10.16 R15.1
N$12  (via drill 0.61)
  Top 0.381: v40.44,33.33 40.44,27.03 41.66,25.81 41.66,25.6 42.67,25.6 42.88,25.4 IC3.24 | v43.28,33.33 43.28,43.69 ANA2.1 | C15.1 41.25,41.45 41.25,43.69 R7.2
  Bottom 0.381: ANA2.1 43.08,43.89 41.45,43.89 R7.2 | v43.28,33.33 v40.44,33.33
N$13  (via drill 0.61)
  Top 0.381: R6.2 39.42,37.39 39.42,34.95 C14.1 39.42,34.75 39.42,32.92 37.8,31.29 37.8,29.26 38.2,28.85 v38.2,23.77 | v43.69,23.77 43.69,25.2 IC3.23
  Bottom 0.381: ANA1.1 41.25,37.39 39.42,37.39 R6.2 | v38.2,23.77 v43.69,23.77
N$14  (via drill 0.61)
  Top 0.508: v20.93,31.09 20.93,33.53 D5.C
  Bottom 0.508: v20.93,31.09 17.88,31.09 R14.1
N$15  (via drill 0.61)
  Top 0.254: v38.81,29.67 38.81,25.2 39.22,24.79 39.22,22.15 41.25,22.15 IC3.27
  Bottom 0.254: v38.81,29.67 39.22,29.26 42.06,29.26 42.67,28.65 55.88,28.65 J2.1
N$16  (via drill 0.61)
  Top 0.254: v39.01,17.48 39.01,18.9 39.42,19.3 39.42,21.34 41.25,21.34 IC3.28 | v36.17,12.6 v36.17,17.48 | v57.3,12.39 57.3,16.87 58.52,18.09 58.52,28.45 J2.2
  Bottom 0.254: v36.17,17.48 v39.01,17.48 | v36.17,12.6 51.82,12.6 52.02,12.39 53.65,12.39 53.85,12.6 54.25,12.6 54.46,12.39 v57.3,12.39
N$17  (via drill 0.61)
  Top 0.254: v46.94,22.15 46.94,25.2 IC3.19 | J2.3 v60.96,22.15
  Bottom 0.254: v46.94,22.15 47.35,22.55 60.55,22.55 v60.96,22.15
N$18  (via drill 0.61)
  Top 0.508: IC2.1 13.01,22.15 13.01,19.1 12.8,19.1 C4.1 12.6,19.1 11.79,19.1 11.58,19.3 v11.58,20.93
  Bottom 0.508: v11.58,20.93 12.7,31.09 R14.2
N$19  (via drill 0.61)
  Top 0.254: v41.45,27.43 42.47,26.42 42.47,26.21 44.3,26.21 44.5,26.01 44.5,25.4 IC3.22 | v36.78,27.43 36.78,20.52 36.17,19.91 36.17,18.69 35.15,17.68 v35.15,11.58 | v60.76,10.97 60.76,11.38 60.55,11.58 60.55,19.3 v60.96,19.71 | v63.6,19.71 63.6,28.45 J2.4
  Bottom 0.254: v36.78,27.43 v41.45,27.43 | v35.15,11.58 36.37,11.58 36.78,11.99 49.58,11.99 51,10.57 51.41,10.57 51.82,10.97 53.44,10.97 53.85,10.57 54.25,10.57 54.66,10.97 v60.76,10.97 | v63.6,19.71 v60.96,19.71
N$20
  Bottom 2.032: F1.1 10.77,58.52 7.11,58.52 5.08,56.49 3.25,56.49 BATT+.1
N$21
  Bottom 2.032: SOLAR+.1 D1.A
N$24
  Top 2.032: D2.C TP2.1
  Bottom 2.032: Q2.D 40.64,72.34 45.72,72.34 D2.C 46.53,72.34 50.8,72.34 L1.2
N$25  (via drill 0.61)
  Top 0.254: v51.61,27.23 51.61,23.77 50.19,23.77 IC3.16 | v69.29,26.01 69.29,12.8 R21.2 | v27.64,2.03 v27.64,4.88 | v67.46,12.8 v67.46,2.03
  Bottom 0.254: v51.61,27.23 53.44,27.23 55.07,25.6 68.89,25.6 v69.29,26.01 | v27.64,4.88 26.01,4.88 25.81,5.08 19.91,5.08 18.69,3.86 17.88,3.86 ISP1.1 | v27.64,2.03 27.84,2.03 28.65,1.22 66.65,1.22 v67.46,2.03 | v67.46,12.8 69.09,12.8 R21.2
N$26  (via drill 0.61)
  Top 0.254: ISP1.5 22.96,3.86 25.4,3.86 v25.4,6.3 RESET.1 | v40.03,18.69 40.03,20.52 41.25,20.52 IC3.29 | R3.2 34.75,20.32 v34.75,18.69 34.75,18.49 33.73,17.48 33.73,6.71 v34.14,6.3
  Bottom 0.254: v34.75,18.69 v40.03,18.69 | v34.14,6.3 v25.4,6.3
N$27  (via drill 0.61)
  Top 0.254: v52.63,29.67 52.63,27.03 52.22,26.62 52.22,22.96 50.19,22.96 IC3.15 | v70.31,29.67 70.31,25.81 69.9,25.4 69.9,14.83 70.71,14.02 v70.71,10.16 v70.71,3.05 | v28.85,2.23 v28.85,7.32
  Bottom 0.254: v52.63,29.67 53.44,30.48 69.49,30.48 v70.31,29.67 | R22.2 v70.71,10.16 | v28.85,7.32 28.45,7.72 24.59,7.72 24.38,7.52 22.35,7.52 21.13,6.3 20.32,6.3 ISP1.4 | v28.85,2.23 29.26,1.83 59.74,1.83 60.96,3.05 v70.71,3.05
N$28  (via drill 0.61)
  Top 0.508: v48.36,48.97 48.36,39.83 IC1.7 | v40.44,49.17 40.44,63.6 40.64,63.8 TP1.1 Q2.G
  Bottom 0.508: v48.36,48.97 48.16,49.17 v40.44,49.17
N$29
  Top 2.032: L1.1 58.52,72.34 58.52,60.96 L4.2
  Bottom 2.032: TP3.1 L4.2 | C2.+ 67.87,74.37 62.38,74.37 60.35,72.34 58.52,72.34 L1.1
N$31
  Top 0.508: LED3.A 63.6,5.08 63.6,10.16 R20.1
N$32  (via drill 0.61)
  Top 0.381: v32.31,49.99 32.31,48.56 31.7,47.95 31.7,45.92 IC4.2
  Bottom 0.381: v32.31,49.99 30.48,49.99 29.46,48.97 28.65,48.97 R10.1 28.45,48.97 26.21,48.97 R13.2
N$33
  Top 0.508: LED4.A 69.29,5.08 69.29,10.16 R21.1
N$34  (via drill 0.61)
  Top 0.508: v74.98,8.33 74.98,5.08 LED5.A | v77.42,8.33 77.42,10.16 R22.1
  Bottom 0.508: v77.42,8.33 v74.98,8.33
N$35  (via drill 0.61)
  Top 0.254: C11.2 55.88,14.02 53.44,14.02 Q6.2 | v47.75,14.02 47.75,16.66 IC3.7
  Bottom 0.254: v47.75,14.02 53.24,14.02 Q6.2
N$36  (via drill 0.61)
  Top 0.254: C12.2 55.88,16.46 53.44,16.46 Q6.1 | IC3.8 49.58,16.66 v49.58,16.46
  Bottom 0.254: v49.58,16.46 53.24,16.46 Q6.1
N$37  (via drill 0.61)
  Top 0.381: IC4.3 30.48,47.55 v30.28,47.75
  Bottom 0.381: v30.28,47.75 32.31,47.75 33.53,48.97 35.56,48.97 | 35.56,48.97 37.39,48.97 R11.2 | 35.56,48.97 R12.2
N$38  (via drill 0.61)
  Top 0.508: 19.71,63.2 R8.1 19.91,63.4 20.73,63.4 20.73,57.3 21.54,56.49 v21.54,35.56 | L3.2 v25.4,35.56 v25.4,39.01
  Bottom 0.508: v25.4,35.56 v21.54,35.56 | v25.4,39.01 27.84,39.01 28.85,40.03 37.39,40.03 37.8,39.62 42.67,39.62 43.08,40.03 60.15,40.03 R31.1
N$39
  Top 0.381: IC4.6 30.48,39.01 29.26,37.8 29.26,37.59 R16.1 29.26,37.39 29.26,34.95 R18.2
N$40  (via drill 0.61)
  Top 0.381: v28.04,40.64 29.06,40.64 IC4.5
  Bottom 0.381: R19.2 v28.04,40.64
N$42
  Top 0.381: IC4.7 31.7,40.44 31.7,37.59 R16.2
  Bottom 0.381: R6.1 36.78,37.39 31.9,37.39 R16.2
N$43
  Bottom 2.032: Q1.D 3.25,15.85 9.55,15.85 9.55,25.81 9.75,26.01 9.75,30.68 3.25,30.68 3.25,36.17 LAST+.1
N$47  (via drill 0.61)
  Top 0.381: 33.12,47.55 33.12,49.38 33.33,49.58 v33.33,51 | 33.12,47.55 33.12,45.92 IC4.1 | v31.09,51 31.09,48.97 R10.2 | v33.73,47.55 33.12,47.55
  Bottom 0.381: v31.09,51 v33.33,51 | R19.1 28.85,45.72 28.96,45.62 | 28.96,45.62 30.07,44.5 36.37,44.5 36.58,44.7 37.39,44.7 38.2,43.89 38.61,43.89 R7.1 | v33.73,47.55 33.12,47.55 32.72,47.14 31.09,47.14 29.67,45.72 29.06,45.72 28.96,45.62
N$50  (via drill 0.61)
  Top 0.254: v46.53,20.73 45.92,20.12 45.92,19.71 41.45,19.71 IC3.30 | v29.87,20.73 29.87,18.69 30.68,17.88 30.68,10.77 30.28,10.36 30.28,6.5 30.48,6.3 J1.1
  Bottom 0.254: v46.53,20.73 46.13,20.32 37.8,20.32 37.39,20.73 v29.87,20.73
N$51  (via drill 0.61)
  Top 0.254: v32.72,14.22 33.12,13.82 33.12,4.47 J1.2 | v42.27,15.04 42.27,17.48 42.47,17.68 42.47,18.69 42.27,18.9 41.45,18.9 IC3.31
  Bottom 0.254: v32.72,14.22 41.45,14.22 v42.27,15.04
N$52  (via drill 0.61)
  Top 0.254: v41.66,6.71 41.25,7.11 41.25,16.46 41.66,16.87 41.66,18.09 41.45,18.09 IC3.32 | J1.3 v35.56,6.71
  Bottom 0.254: v35.56,6.71 v41.66,6.71
N$53  (via drill 0.61)
  Top 0.254: v38.2,8.33 38.2,4.47 J1.4 | v44.3,8.53 44.09,8.74 44.09,13.82 43.28,14.63 43.28,15.24 42.88,15.65 42.88,16.66 IC3.1
  Bottom 0.254: v38.2,8.33 38.81,8.94 43.89,8.94 v44.3,8.53
N$54  (via drill 0.61)
  Top 0.254: v43.69,18.09 43.69,16.66 IC3.2 | J1.5 v40.64,17.07
  Bottom 0.254: v43.69,18.09 42.67,17.07 v40.64,17.07
N$55  (via drill 0.61)
  Top 0.254: v44.7,14.43 44.7,9.35 45.31,8.74 45.31,8.13 43.28,6.1 43.28,4.47 J1.6 | v48.56,18.09 49.99,18.09 IC3.9
  Bottom 0.254: v44.7,14.43 44.7,18.09 v48.56,18.09
N$56  (via drill 0.61)
  Top 0.254: v49.99,6.71 49.99,11.58 50.6,12.19 50.6,15.85 51,16.26 51,18.9 50.19,18.9 IC3.10 | J1.7 v45.72,6.71
  Bottom 0.254: v45.72,6.71 v49.99,6.71
N$57  (via drill 0.61)
  Top 0.254: v48.56,19.3 48.97,19.71 49.99,19.71 IC3.11 | v37.19,9.14 v37.19,19.71 | v48.36,9.14 48.36,4.47 J1.8
  Bottom 0.254: v48.56,19.3 48.16,19.71 v37.19,19.71 | v37.19,9.14 37.59,9.55 45.31,9.55 45.72,9.14 v48.36,9.14
N$58
  Top 0.381: R27.2 67.87,45.11 67.87,47.55 R24.2
  Bottom 0.381: R25.1 69.7,47.55 68.07,47.55 R24.2
N$60  (via drill 0.61)
  Top 2.032: R12.1 TP4.1 34.95,59.74 34.95,60.96 R9.2 | v54.66,54.46 54.66,60.96 L4.1
  Bottom 2.032: v54.66,54.46 52.22,54.46 C3.+ | L4.1 R9.2
N$64
  Top 0.381: R34.2 67.87,37.59 67.87,39.83 R31.2
  Bottom 0.381: R26.1 69.7,40.03 68.07,40.03 R31.2
SOLARDUENN  (via drill 0.61)
  Top 0.508: v57.91,49.38 57.91,47.75 R4.2 | v60.35,49.38 60.35,47.75 R24.1 | v35.56,68.07 R17.1 | v56.49,68.07 56.69,67.87 56.69,62.99 56.49,62.79 v56.49,49.58
  Bottom 0.508: v60.35,49.38 v57.91,49.38 57.91,49.58 v56.49,49.58 | v56.49,68.07 v35.56,68.07
SOLPLUS  (via drill 0.61)
  Top 2.032: v35.56,77.42 R17.2 | Q2.S v40.64,77.42
  Bottom 2.032: v40.64,77.42 v35.56,77.42 34.95,76.61 34.14,75.79 31.09,75.79 C1.+ 30.48,74.98 28.45,74.98 27.23,76.2 D1.C
V12  (via drill 0.61)
  Top 2.032: R13.1 26.01,56.69 26.01,58.93 TP5.1 27.03,59.13 27.23,59.33 27.23,60.96 R9.1 | v22.55,60.96 22.55,66.24 19.71,66.24 R8.2 | v6.91,18.49 9.55,21.13 9.55,25.81 9.75,26.01 9.75,31.29 10.77,32.31 10.77,33.53 D5.A 10.77,34.54 10.77,43.08 F1.2 | v23.37,45.72 v23.37,56.49
  Bottom 2.032: R9.1 v22.55,60.96 | v6.91,18.49 3.25,18.49 Q1.S | v23.37,56.49 26.01,56.49 R13.1 | v23.37,45.72 20.93,45.72 20.73,45.92 18.49,45.92 17.07,44.5 13.41,44.5 12.19,43.28 10.97,43.28 F1.2
V+
  Top 0.508: C8.1 34.75,41.05 33.12,41.05 33.12,40.64 IC4.8 33.12,40.44 33.12,39.01 33.33,38.81 33.33,38.61 33.53,38.41 33.53,35.76 33.12,35.36 33.12,32.51 L3.1
VCC  (via drill 0.61)
  Top 0.381: IC2.3 17.48,22.15 17.48,19.1 17.68,19.1 C5.1 17.88,19.1 20.32,19.1 C7.1 v20.32,22.55 VCC.1 L2.1 | 46.94,16.66 46.94,15.85 47.14,15.65 47.14,14.83 45.92,13.61 45.92,12.8 C6.1 45.92,12.6 v45.92,10.16 | 46.94,16.66 46.94,17.48 46.53,17.88 45.72,17.88 45.31,17.48 IC3.4 | v31.29,22.35 31.29,20.32 | 31.29,20.32 v31.29,10.16 | 31.29,20.32 R3.1 | 46.94,16.66 IC3.6
  Bottom 0.381: v31.29,22.35 25.81,22.35 25.4,22.76 20.52,22.76 v20.32,22.55 | R15.2 v31.29,10.16 v45.92,10.16
VS  (via drill 0.61)
  Top 0.508: v49.58,38.2 49.58,39.62 IC1.6 | v52.22,38.2 52.43,38.41 53.85,38.41 C13.1 54.05,38.41 54.86,38.41 55.07,38.61 55.07,47.55 R4.1
  Bottom 0.508: v52.22,38.2 v49.58,38.2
